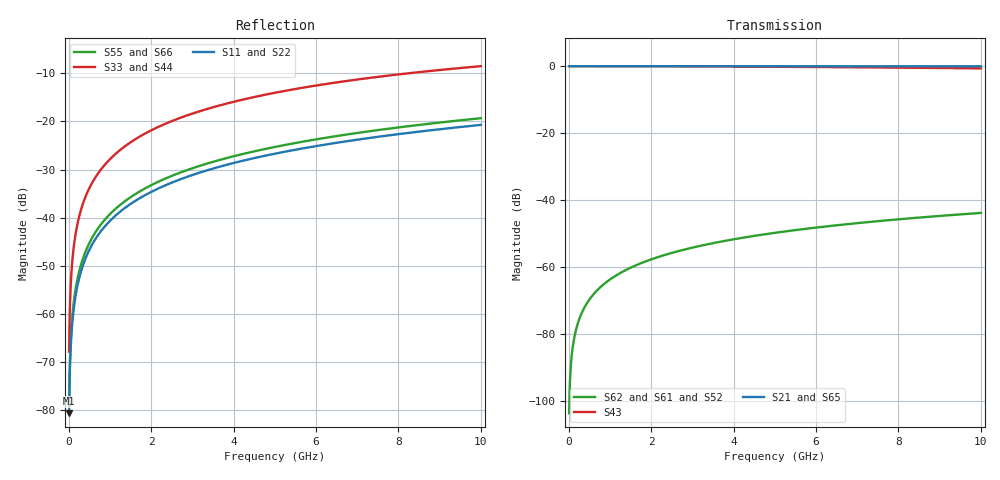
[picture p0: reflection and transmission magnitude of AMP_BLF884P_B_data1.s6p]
! Created Thu Nov 14 13:29:56 2013
# ghz S ma R 50
! 6 Port Network Data from SP1.SP block
! freq  magS11  angS11  magS12  angS12  magS13  angS13  magS14  angS14
!  magS15  angS15  magS16  angS16
!  magS21  angS21  magS22  angS22
!  magS23  angS23  magS24  angS24  magS25  angS25  magS26  angS26
!  magS31  angS31  magS32  angS32  magS33  angS33  magS34  angS34
!  magS35  angS35  magS36  angS36
!  magS41  angS41  magS42  angS42
!  magS43  angS43  magS44  angS44  magS45  angS45  magS46  angS46
!  magS51  angS51  magS52  angS52  magS53  angS53  magS54  angS54
!  magS55  angS55  magS56  angS56
!  magS61  angS61  magS62  angS62
!  magS63  angS63  magS64  angS64  magS65  angS65  magS66  angS66
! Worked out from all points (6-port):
!   1000 points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, 10 MHz to 10 GHz, reference 50 ohm
!   strongest paths, dB at 10 MHz, 2.51 GHz, 5.01 GHz, 7.51 GHz, 10 GHz:
!     S21: 0.0, 0.0, 0.0, 0.0, 0.0
!     S65: 0.0, 0.0, 0.0, 0.0, -0.1
!     S43: 0.0, 0.0, -0.2, -0.4, -0.7
!     S62: -103.8, -55.8, -49.8, -46.3, -43.9
!     S61: -103.8, -55.8, -49.8, -46.3, -43.9
!     S52: -103.8, -55.8, -49.8, -46.3, -43.9
!   lowest |S11| = -80.7 dB at 10 MHz (marker M1), VSWR 1.00, Z = 50 + j0.00925 ohm
!   |S11| at or under -10 dB: start of sweep to end of sweep
